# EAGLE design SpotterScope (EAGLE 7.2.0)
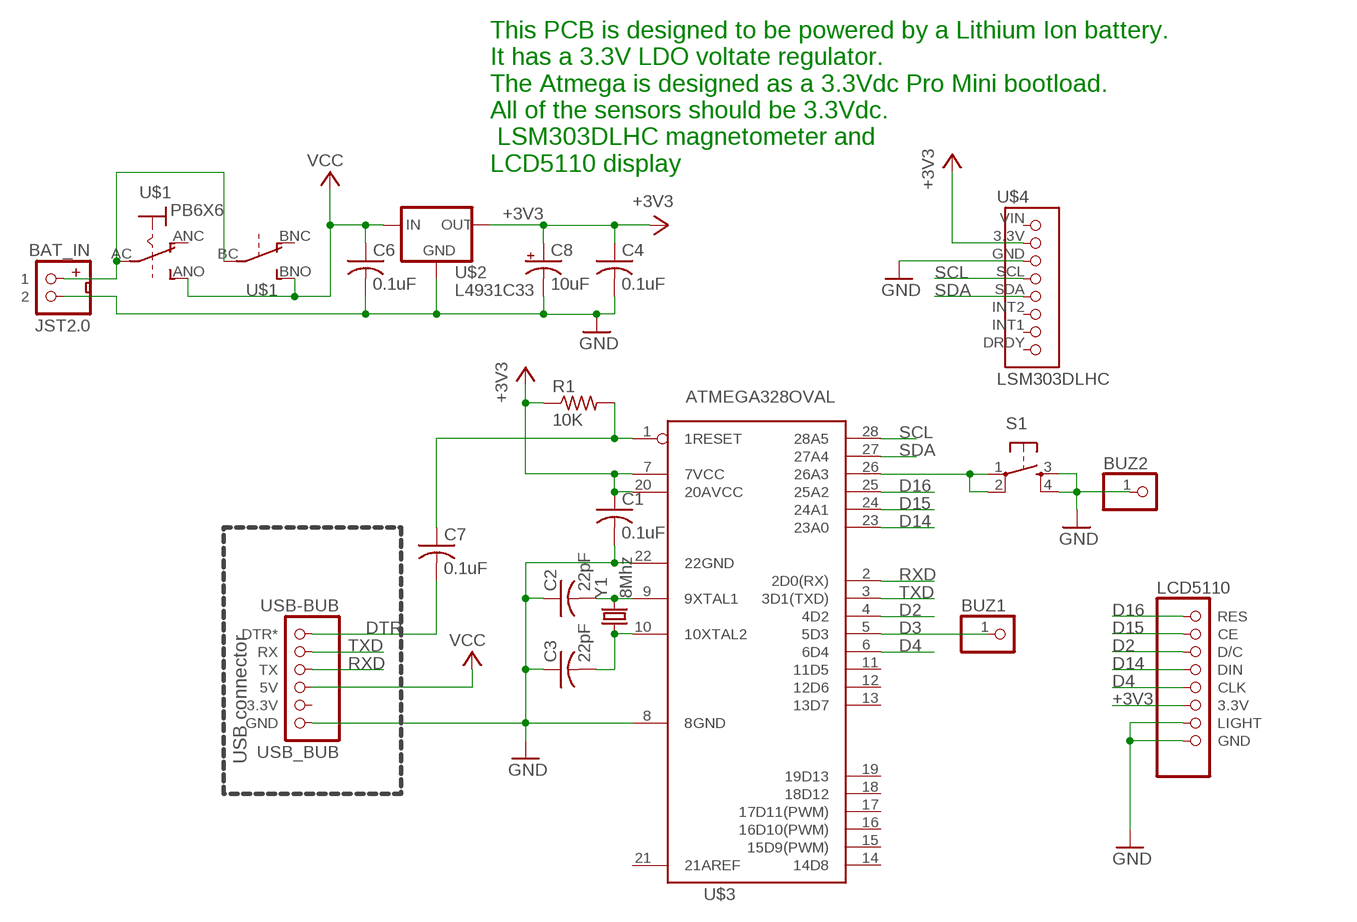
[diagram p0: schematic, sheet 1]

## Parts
BAT_IN  JST2.0  [JST2.0]
BUZ1  PINHD-1X1  [1X01]
BUZ2  PINHD-1X1  [1X01]
C1  0.1uF  C-US050-024X044  [C050-024X044]
C2  22pF  C-US025-025X050  [C025-025X050]
C3  22pF  C-US025-025X050  [C025-025X050]
C4  0.1uF  C-US025-025X050  [C025-025X050]
C6  0.1uF  C-US025-025X050  [C025-025X050]
C7  0.1uF  C-US075-042X103  [C075-042X103]
C8  10uF  CPOL-USE2.5-5V  [E2,5-4R]
LCD5110  LCD5110_1TOP  [LCD5110T1]
R1  10K  R-US_0207/5V  [0207/5V]
S1  TAC_SWITCHPTH  [TACTILE-PTH]
U$1  PB6X6  [PB6X6]
U$2  L4931C33  [TO92-INLINE]
U$3  ATMEGA328OVAL  [DIL28-3]
U$4  LSM303DLHC  [LSM303DLHC]
USB-BUB  USB_BUB  [USB_BUB]
Y1  8Mhz  CRYSTALTC38H  [TC38H]

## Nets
+3V3: C1.1 C4.1 C8.+ LCD5110.3.3V R1.1 U$2.1(OUT) U$3.7(7VCC) U$3.20(20AVCC) U$4.3.3V
D2: LCD5110.D/C U$3.4(4D2)
D3: BUZ1.1 U$3.5(5D3)
D4: LCD5110.CLK U$3.6(6D4)
D14: LCD5110.DIN U$3.23(23A0)
D15: LCD5110.CE U$3.24(24A1)
D16: LCD5110.RES U$3.25(25A2)
DTR: C7.2 USB-BUB.DTR*
GND [power]: BAT_IN.2 BUZ2.1 C1.2 C2.1 C3.1 C4.2 C6.2 C8.- LCD5110.GND LCD5110.LIGHT S1.3 S1.4 U$2.2(GND) U$3.8(8GND) U$3.22(22GND) U$4.GND USB-BUB.GND
N$1: S1.1 S1.2 U$3.26(26A3)
N$2: BAT_IN.1 U$1.AC(P) U$1.BC(P)
N$6: C3.2 U$3.10(10XTAL2) Y1.1
N$7: C2.2 U$3.9(9XTAL1) Y1.2
RESET: C7.1 R1.2 U$3.1(1RESET)
RXD: U$3.2(2D0(RX)) USB-BUB.TX
SCL: U$3.28(28A5) U$4.SCL
SDA: U$3.27(27A4) U$4.SDA
TXD: U$3.3(3D1(TXD)) USB-BUB.RX
VCC: C6.1 U$1.ANO(S) U$1.BNO(S) U$2.3(IN) USB-BUB.5V
Unconnected: U$1.ANC(O) U$1.BNC(O) U$3.11(11D5) U$3.12(12D6) U$3.13(13D7) U$3.14(14D8) U$3.15(15D9(PWM)) U$3.16(16D10(PWM)) U$3.17(17D11(PWM)) U$3.18(18D12) U$3.19(19D13) U$3.21(21AREF) U$4.DRDY U$4.INT1 U$4.INT2 U$4.VIN USB-BUB.3.3V

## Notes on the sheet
- This PCB is designed to be powered by a Lithium Ion battery. 
  It has a 3.3V LDO voltate regulator. 
  The Atmega is designed as a 3.3Vdc Pro Mini bootload.
  All of the sensors should be 3.3Vdc.
   LSM303DLHC magnetometer and
  LCD5110 display
- USB connector

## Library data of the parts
BAT_IN = MTS_Custom:JST2.0
BUZ1 BUZ2 = pinhead:PINHD-1X1: PIN HEADER
C1-C4 C6 C7 = rcl:C-US: CAPACITOR, American symbol
C8 = rcl:CPOL-US: POLARIZED CAPACITOR, American symbol
LCD5110 = MTS_Custom:LCD5110_1
R1 = rcl:R-US_: RESISTOR, American symbol
S1 = SparkFun:TAC_SWITCH: Momentary Switch Button commonly used for reset or general input. Spark Fun Electronics SKU : COM-00097
U$1 = MTS_Custom:PB6X6: Pushbutton 6mm x 6mm DPDT. 0.5A, 50V should be the same for momentary and latching.
U$2 = MTS_Custom:L4931C33: Voltage Regulator 3.3Vdc LDO (0.4V)
U$3 = MTS_Custom:ATMEGA328
U$4 = MTS_Custom:LSM303DLHC: 3 Axis Magnetometer and 3 Axis Accelerometer Module
USB-BUB = MTS_Custom:USB_BUB
Y1 = crystal:CRYSTAL: CRYSTAL; OC_FARNELL: unknown; OC_NEWARK: unknown

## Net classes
0 default: width 0.305 mm
1 power: width 0.6 mm, clearance 0.3 mm

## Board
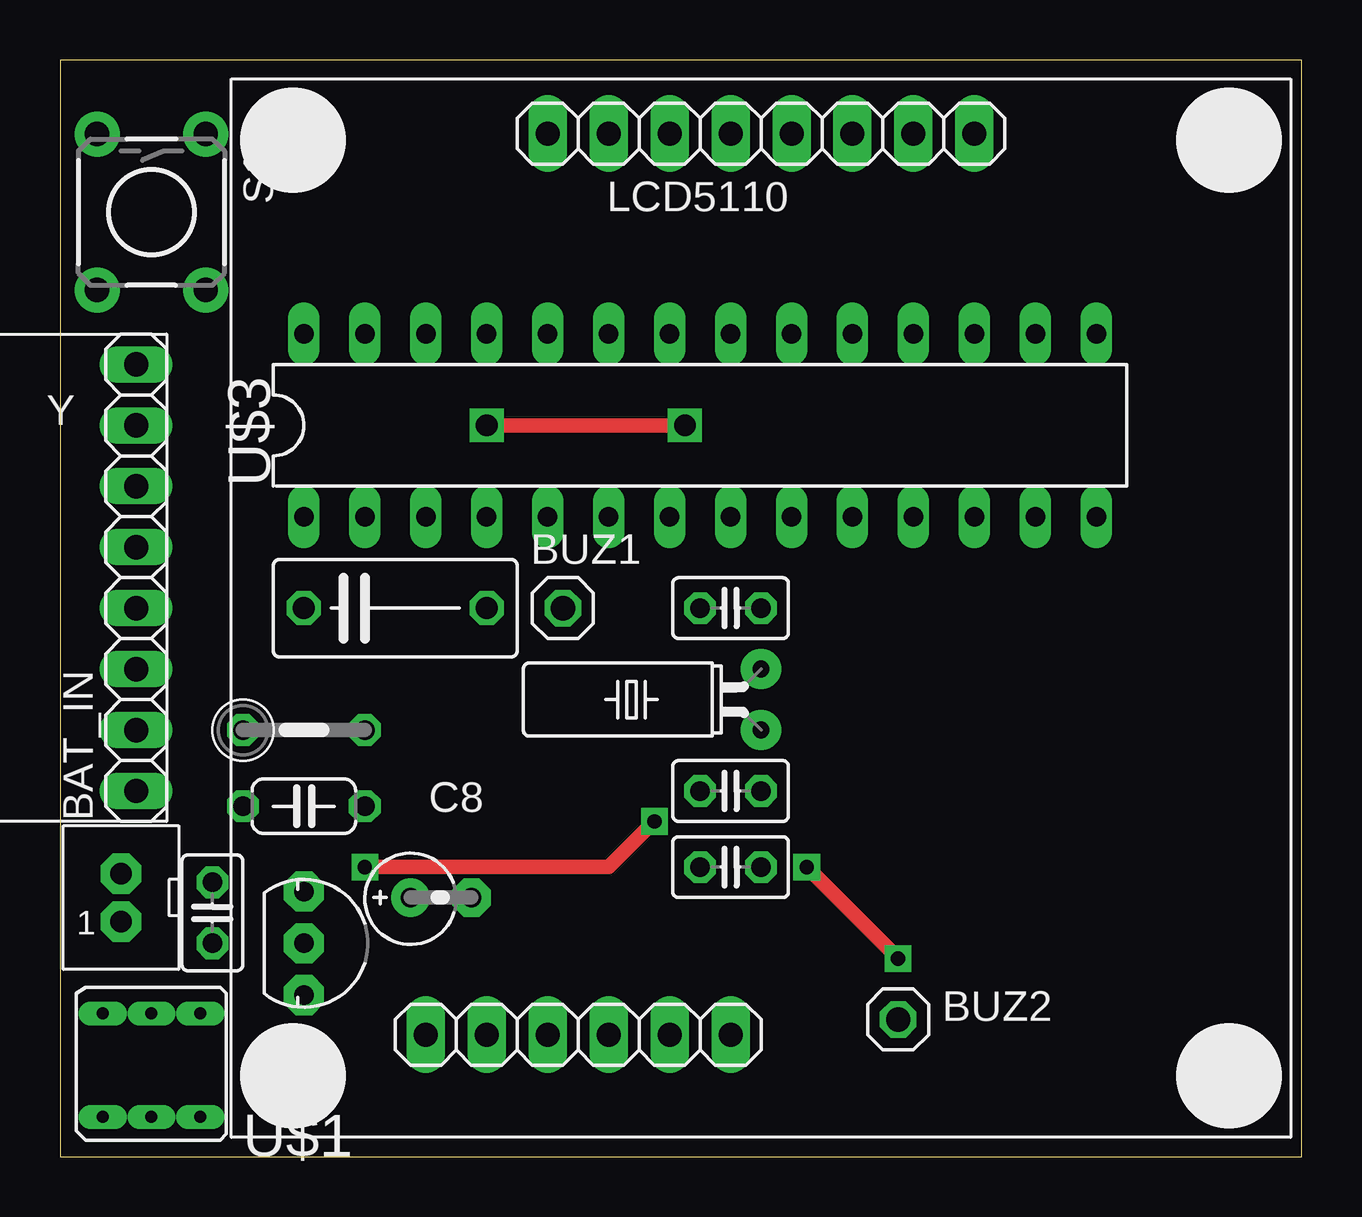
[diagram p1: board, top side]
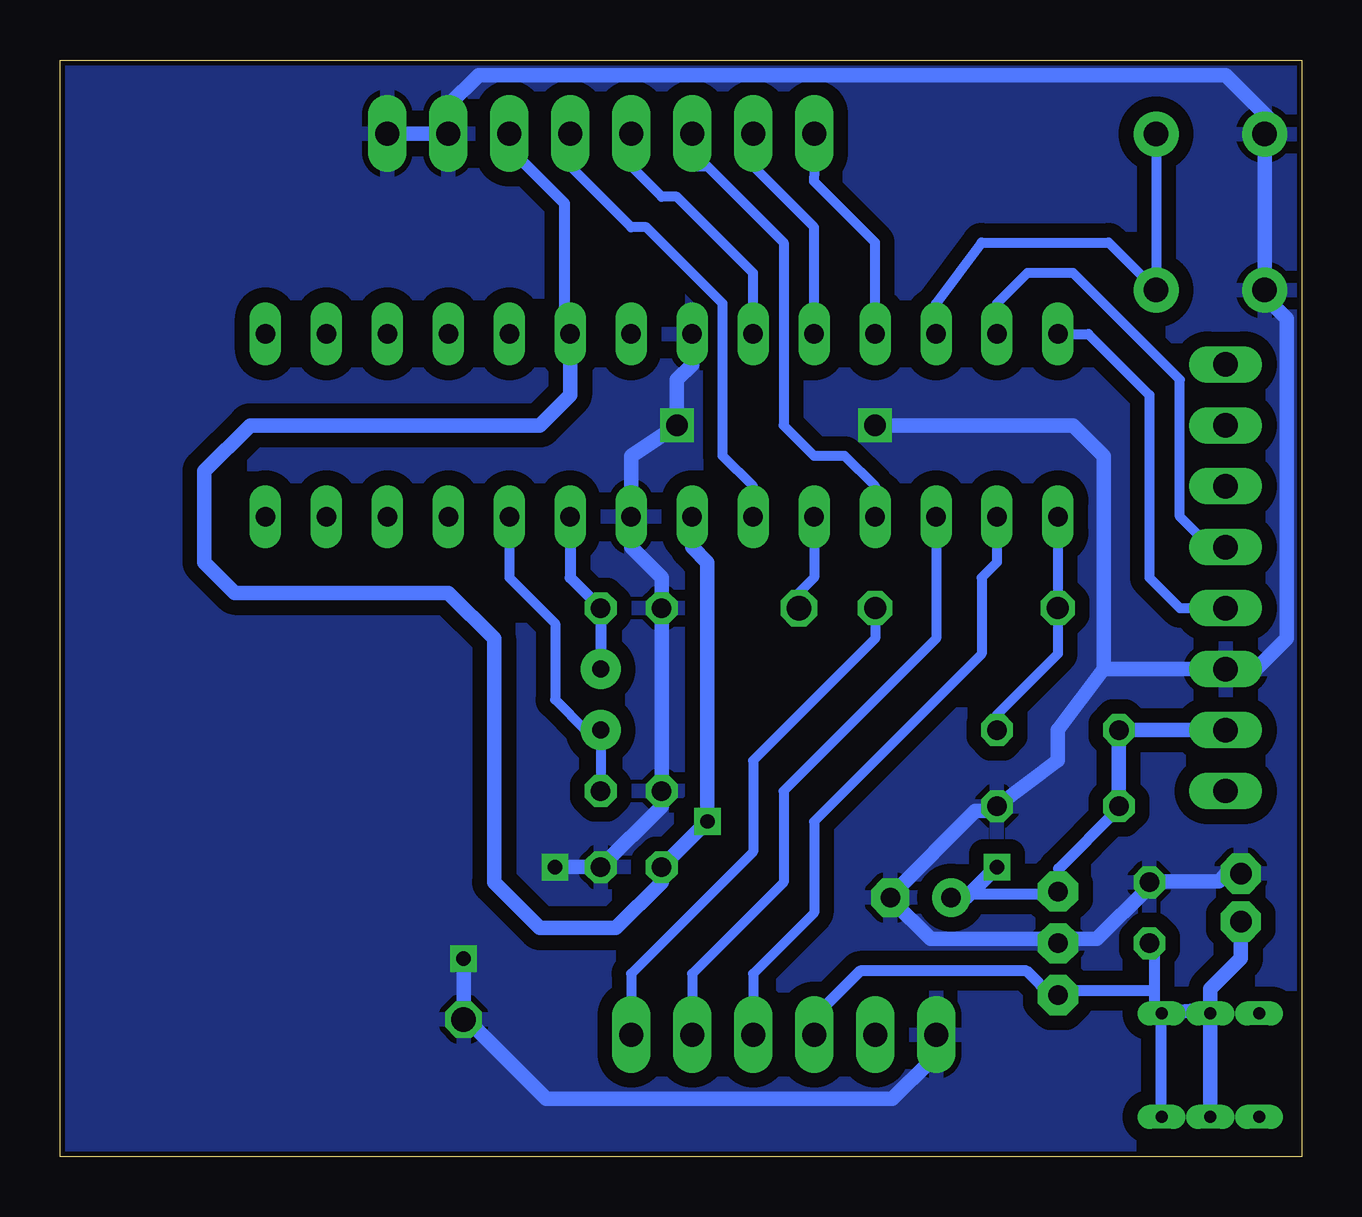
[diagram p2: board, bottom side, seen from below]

Size 51.74 x 45.71 mm. Coordinates in mm from the lower left corner, seen from the top.
Outline: 0,0 51.74,0 51.74,45.71 0,45.71 0,0
Copper layers (1*16): Top 0.035mm / dielectric 1.5mm / Bottom 0.035mm
Design rules "MTS": minimum track width 18mil, minimum drill 12mil, track to track 24mil, track to pad 24mil, pad to pad 6mil, via to via 6mil, smd to smd 0mil, copper to edge 8mil, drill to drill 10mil, minimum pad ring 10mil, minimum via ring 10mil, stop-mask expansion 2mil, vias tented up to drill 25mil, thermal gap 10mil

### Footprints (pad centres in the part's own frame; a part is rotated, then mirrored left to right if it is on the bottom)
JST2.0 = drill 0.9 pad 1.676 octagon: 1 0,-1; 2 0,1
1X01 = drill 1.016 octagon: 1 0,0
C050-024X044 = drill 0.813 octagon: 1 -2.54,0; 2 2.54,0
C025-025X050 = drill 0.813 octagon: 1 -1.27,0; 2 1.27,0
C075-042X103 = drill 0.914 octagon: 1 -3.81,0; 2 3.81,0
E2,5-4R = drill 0.813 pad 1.6: + -1.27,0 | drill 0.813 pad 1.6 octagon: - 1.27,0
LCD5110T1 = drill 1 pad 1.6 long: 3.3V 3.81,19.78; CE -6.35,19.78; CLK 1.27,19.78; D/C -3.81,19.78; DIN -1.27,19.78; GND 8.89,19.78; LIGHT 6.35,19.78; RES -8.89,19.78
0207/5V = drill 0.813 octagon: 1 -2.54,0; 2 2.54,0
TACTILE-PTH = drill 1.016 pad 1.88: 1 -3.251,2.261; 2 3.251,2.261; 3 -3.251,-2.261; 4 3.251,-2.261
PB6X6 = drill 0.5 pad 0.813 long: AC -2.159,0; ANC -2.159,-2.032; ANO -2.159,2.032; BC 2.159,0; BNC 2.159,-2.032; BNO 2.159,2.032
TO92-INLINE = drill 0.813 pad 1.676 octagon: 1 -2.159,0; 2 0,0; 3 2.159,0
DIL28-3 = drill 0.813 long: 1 -16.51,-3.81; 2 -13.97,-3.81; 3 -11.43,-3.81; 4 -8.89,-3.81; 5 -6.35,-3.81; 6 -3.81,-3.81; 7 -1.27,-3.81; 8 1.27,-3.81; 9 3.81,-3.81; 10 6.35,-3.81; 11 8.89,-3.81; 12 11.43,-3.81; 13 13.97,-3.81; 14 16.51,-3.81; 15 16.51,3.81; 16 13.97,3.81; 17 11.43,3.81; 18 8.89,3.81; 19 6.35,3.81; 20 3.81,3.81; 21 1.27,3.81; 22 -1.27,3.81; 23 -3.81,3.81; 24 -6.35,3.81; 25 -8.89,3.81; 26 -11.43,3.81; 27 -13.97,3.81; 28 -16.51,3.81
LSM303DLHC = drill 1.016 long: 3.3V -2.54,5.08; DRDY -2.54,-10.16; GND -2.54,2.54; INT1 -2.54,-7.62; INT2 -2.54,-5.08; SCL -2.54,0; SDA -2.54,-2.54; VIN -2.54,7.62
USB_BUB = drill 1 pad 1.6 long: 3.3V -3.81,0; 5V -1.27,0; DTR* 6.35,0; GND -6.35,0; RX 3.81,0; TX 1.27,0
TC38H = drill 0.7 pad 1.676: 1 -1.27,0; 2 1.27,0

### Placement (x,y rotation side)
BAT_IN  2.54,10.79 0 top
BUZ1  20.95,22.86 0 top
BUZ2  34.92,5.71 0 top
C1  10.16,14.61 0 top
C2  27.94,22.86 0 top
C3  27.94,15.24 0 top
C4  27.94,12.06 0 top
C6  6.35,10.16 90 top
C7  13.97,22.86 0 top
C8  15.88,10.79 0 top
LCD5110  29.21,22.86 0 top
R1  10.16,17.78 0 top
S1  3.81,39.37 270 top
U$1  3.81,3.81 270 top
U$2  10.16,8.89 270 top
U$3  26.67,30.48 0 top
U$4  0.64,22.86 180 top
USB-BUB  21.59,5.08 0 top
Y1  29.21,19.05 90 top

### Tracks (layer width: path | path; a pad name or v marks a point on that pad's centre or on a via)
+3V3  (via drill 0.6)
  Top 0.61: v12.7,12.06 22.86,12.06 v24.77,13.97
  Bottom 0.457: U$3.20 30.72,34.4 30.72,39.74 32.85,41.87 32.85,42.41 LCD5110.3.3V | C8.+ 14.4,10.94 10.4,10.94 U$2.1 10.13,11.2 10.13,12 7.73,14.4 C1.1
  Bottom 0.61: C1.1 R1.1 U$4.3.3V | U$3.7 25.4,25.4 24.77,24.77 v24.77,13.97 C4.1 26.67,11.43 28.57,9.53 31.75,9.53 33.66,11.43 33.66,21.59 35.56,23.5 44.45,23.5 45.72,24.77 45.72,28.57 43.81,30.48 31.75,30.48 30.48,31.75 U$3.20 | C8.+ 13.97,10.79 v12.7,12.06
D2
  Bottom 0.406: LCD5110.D/C 25.4,41.27 24.77,41.27 21.59,38.1 21.59,30.48 20.32,29.21 19.05,29.21 17.78,27.94 U$3.4
D3
  Bottom 0.406: U$3.5 20.32,24.13 20.95,23.5 BUZ1.1
D4
  Bottom 0.406: U$3.6 22.86,27.94 24.13,29.21 24.13,35.56 27.3,38.73 27.94,38.73 30.48,41.27 LCD5110.CLK
D14
  Bottom 0.406: U$3.23 22.86,36.83 26.04,40.01 26.67,40.01 27.94,41.27 LCD5110.DIN
D15
  Bottom 0.406: U$3.24 20.32,38.73 22.86,41.27 LCD5110.CE
D16
  Bottom 0.406: U$3.25 17.78,38.1 20.32,40.64 20.23,42.55 LCD5110.RES
DTR
  Bottom 0.406: C7.2 17.78,21.59 22.86,16.51 22.86,12.7 27.94,7.62 USB-BUB.DTR*
GND  (via drill 0.6 pad 0.81, 0.9)
  Top 0.61: v17.78,30.48 v26.04,30.48 | v31.11,12.06 v34.92,8.26
  Bottom 0.6: U$3.8 27.94,25.4 26.67,24.13 C2.1 | 34.94,5.97 BUZ2.1 34.67,5.6 31.47,2.4 17.07,2.4 15.47,4 15.47,5.07 USB-BUB.GND | BAT_IN.2 2.67,11.73 3.2,11.73 3.47,11.47 6.13,11.47 C6.2 6.4,11.2 8.53,9.07 10.13,9.07 U$2.2 10.4,9.07 15.47,9.07 17.07,10.67 C8.- 17.07,10.94 13.6,14.4 12.8,14.4 C1.2
  Bottom 0.61: U$3.22 25.4,33.02 26.04,32.38 v26.04,30.48 27.94,29.21 U$3.8 | LCD5110.GND LCD5110.LIGHT 35.56,43.81 34.29,45.09 3.17,45.09 1.27,43.18 1.27,42.9 S1.3 S1.4 1.55,35.84 0.64,34.92 0.64,21.59 1.91,20.32 U$4.GND 8.26,20.32 | v17.78,30.48 9.53,30.48 8.26,29.21 8.26,20.32 | C1.2 10.16,16.51 10.16,17.78 8.26,20.32 | C2.1 C3.1 26.67,14.61 C4.2 v31.11,12.06 | v34.92,8.26 BUZ2.1
  pour Bottom: 0,0 0,45.72 52.07,45.72 52.07,0
N$1
  Bottom 0.406: S1.1 S1.2 8.05,38.1 13.34,38.1 15.24,35.56 U$3.26
N$2
  Bottom 0.61: U$1.BC U$1.AC 3.81,6.99 2.54,8.26 BAT_IN.1
N$6
  Bottom 0.406: U$3.10 33.02,24.13 31.11,22.23 31.11,19.05 29.84,17.78 Y1.1 C3.2
N$7
  Bottom 0.457: U$3.9 30.48,24.13 C2.2 Y1.2
RESET
  Bottom 0.406: U$3.1 C7.1 10.16,20.95 12.7,18.41 R1.2
RXD
  Bottom 0.406: U$3.2 12.7,24.77 13.34,24.13 13.34,20.95 20.32,13.97 20.32,10.16 22.86,7.62 USB-BUB.TX
SCL
  Bottom 0.406: U$3.28 8.89,34.29 6.35,31.75 6.35,24.13 5.08,22.86 U$4.SCL
SDA
  Bottom 0.406: U$4.SDA 3.81,25.4 5.08,26.67 5.08,32.38 9.53,36.83 11.43,36.83 12.7,35.56 U$3.27
TXD
  Bottom 0.406: U$3.3 15.24,21.59 21.59,15.24 21.59,11.43 25.4,7.62 USB-BUB.RX
VCC
  Bottom 0.457: U$1.BNO 5.87,1.87 5.87,5.87 U$1.ANO 6.13,5.87 6.13,6.93 | 6.13,6.93 6.13,8.8 C6.1 | USB-BUB.5V 20.27,5.33 20.27,5.87 18.4,7.73 11.47,7.73 10.4,6.67 U$2.3 10.13,6.93 6.13,6.93
  Bottom 0.61: 4.45,6.1 U$1.ANO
